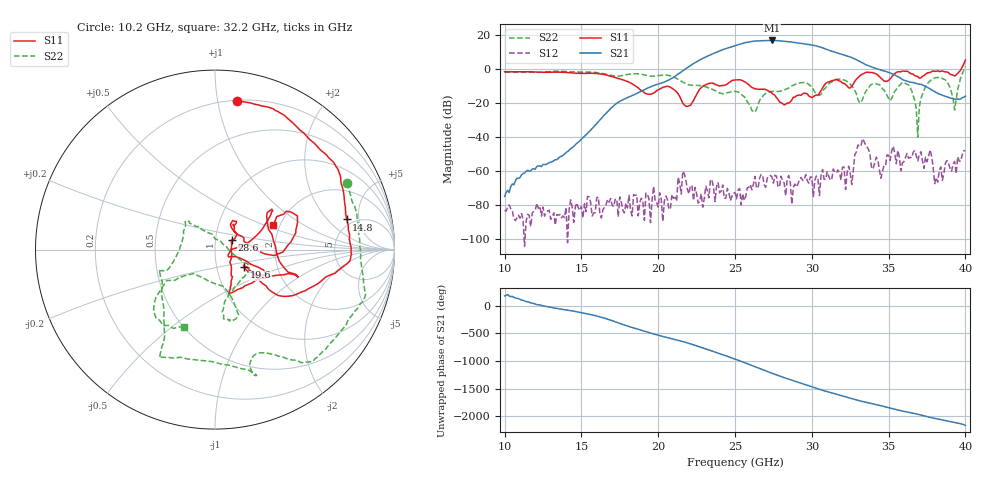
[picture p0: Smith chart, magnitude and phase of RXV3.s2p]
!Keysight Technologies,M9808A,MY58100618,A.14.70.03
!Date: Monday, February 27, 2023 13:44:15
!Correction: S11(Cdelta 2-Port  )
!S21(Cdelta 2-Port  )
!S12(Cdelta 2-Port  )
!S22(Cdelta 2-Port  )
!S2P File: Measurements: S11, S21, S12, S22:
# Hz S  RI  R 50
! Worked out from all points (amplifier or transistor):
!   301 points, 10 GHz to 40 GHz, reference 50 ohm
!   highest |S21| = 17.0 dB at 27.4 GHz (marker M1)
!   |S21| within 3 dB of that: 25.02 GHz to 30.19 GHz (5.166 GHz wide, 18.7 % of centre)
!   unconditionally stable (mu >= 1): start of sweep to 39.72 GHz
!   at 15 GHz: K = 90069.79, MAG = -32.7 dB, |S12| = -81.0 dB
!   at 25 GHz: K = 319.78, MAG = 15.3 dB, |S12| = -72.8 dB
!   at 40 GHz: K = 1013.03, MSG = 16.1 dB, |S12| = -48.2 dB
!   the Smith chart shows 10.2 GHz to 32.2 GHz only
!   S11 on the Smith chart (normalised r, x): 10.2 GHz: 0.21, +1.14; 14.8 GHz: 4.37, +3.39; 19.6 GHz: 1.35, -0.27; 28.6 GHz: 1.20, +0.13; 32.2 GHz: 1.85, +0.57
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1e10  0.0671 0.8387  -0.000177 2.37e-06  1.17e-05 6.89e-05  0.7136 0.4308
1.02e10  0.122 0.8268  -0.000245 -0.000105  3.29e-06 -8.66e-05  0.7333 0.3713
1.48e10  0.7339 0.1683  -0.0028 -0.00647  8.03e-05 3.91e-06  0.6656 -0.498
1.5e10  0.7432 0.1101  -0.00502 -0.00701  -8.6e-05 2.18e-05  0.631 -0.5343
1.96e10  0.1618 -0.0976  -0.2457 -0.1967  -5.05e-06 -0.000136  -0.0611 -0.619
2e10  0.2108 -0.1278  -0.3615 -0.041  -4.25e-06 -8.48e-05  -0.228 -0.6045
2.27e10  0.2404 0.0873  1.703 -0.7641  4.64e-05 0.000115  -0.3074 -0.1179
2.37e10  0.2913 0.207  -1.4 -2.699  7.54e-05 -9.97e-05  -0.2269 -0.0576
2.44e10  0.344 -0.0227  -4.038 0.3935  -0.000143 6.13e-05  -0.1738 0.0843
2.5e10  0.457 -0.1491  -2.003 4.545  0.000135 -0.000187  -0.1598 0.1526
2.56e10  0.4076 -0.134  3.57 4.735  1.7e-05 0.000132  -0.0861 0.1283
2.62e10  0.2079 -0.1852  6.517 -1.55  -0.00041 -2.64e-05  0.0288 0.0485
2.68e10  0.0827 -0.2422  1.404 -6.799  -0.000732 2.08e-05  0.145 -0.0595
2.74e10  0.0897 -0.1761  -5.435 -4.495  0.000585 0.000337  0.19 -0.1094
2.79e10  0.0826 -0.0701  -6.734 1.347  -0.000333 7.41e-05  0.1405 -0.1736
2.86e10  0.0945 0.0538  -1.256 6.274  0.000118 -0.000445  0.0539 -0.288
2.94e10  0.1174 0.1447  5.01 2.727  -0.000492 -0.000193  0.0792 -0.3972
3e10  0.1108 0.0951  4.679 -2.272  -0.000638 -0.000104  0.1013 -0.2839
3.11e10  0.4226 0.0425  -1.961 -3.084  -0.000509 0.000476  -0.2968 -0.2149
3.22e10  0.3249 0.1357  -2.239 1.197  -0.000256 0.000117  -0.1749 -0.4305
3.5e10  0.448 -0.1414  0.5703 -0.5693  -0.00058 -0.00281  -0.00286 -0.1377
4e10  1.04 -1.563  0.1589 -0.0177  -0.0038 0.000829  0.5842 -1.076
